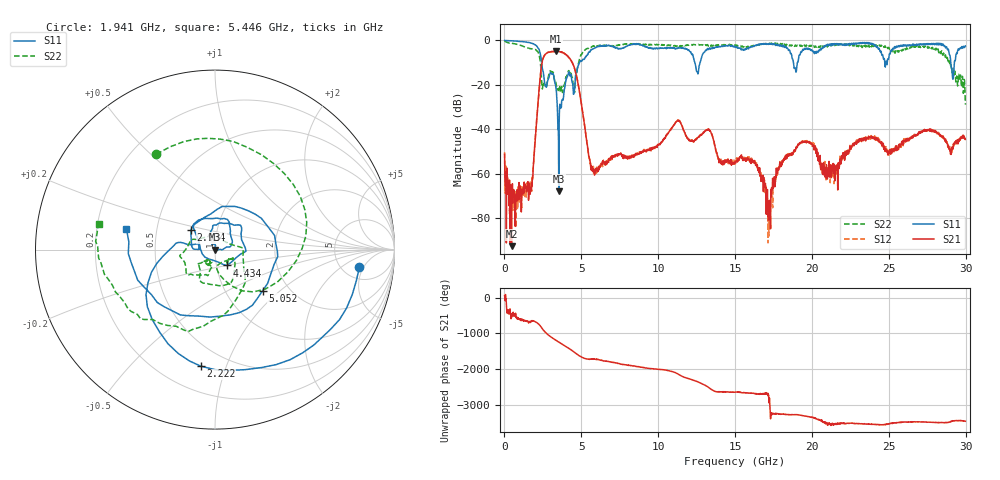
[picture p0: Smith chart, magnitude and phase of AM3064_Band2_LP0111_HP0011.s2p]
# Hz S DB R 50.0
!freq dBS11 angS11 dBS21 angS21 dBS12 angS12 dBS22 angS22
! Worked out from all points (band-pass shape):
!   1600 points, 10 MHz to 29.98 GHz, reference 50 ohm
!   highest |S21| = -4.79 dB at 3.328 GHz (marker M1); lowest = -92.8 dB at 459.8 MHz (marker M2)
!   |S21| within 3 dB of the highest: 2.53 GHz to 4.202 GHz (1.671 GHz wide, 49.6 % of centre)
!   lowest |S11| = -68.0 dB at 3.534 GHz (marker M3), VSWR 1.00, Z = 50 + j0.0316 ohm
!   |S11| at or under -10 dB: 2.416 GHz to 4.88 GHz (2.464 GHz wide, 67.5 % of centre); 12.38 GHz to 12.72 GHz (343.5 MHz wide, 2.74 % of centre); 18.8 GHz to 19.05 GHz (252.6 MHz wide, 1.33 % of centre)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
!   |S22| runs from -28.9 to -0.2 dB; largest |S21 - S12| = 0.023
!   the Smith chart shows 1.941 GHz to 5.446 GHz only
!   S11 on the Smith chart (normalised r, x): 1.941 GHz: 7.17, -4.08; 2.222 GHz: 0.36, -0.82; 2.934 GHz: 0.75, +0.17; 4.434 GHz: 1.12, -0.20; 5.052 GHz: 1.48, -0.78; 5.446 GHz: 0.33, +0.10
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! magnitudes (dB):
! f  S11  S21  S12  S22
! 10 MHz  0.0  -51.3  -50.5  -0.2
! 459.8 MHz  -0.2  -92.8  -71.3  -1.2
! 1.697 GHz  -1.1  -66.1  -66.4  -3.7
! 1.941 GHz  -1.8  -50.4  -50.9  -4.1
! 2.222 GHz  -3.7  -24.9  -24.8  -5.8
! 2.934 GHz  -15.3  -5.3  -5.2  -14.1
! 3.328 GHz  -20.4  -4.8  -4.9  -18.4
! 3.534 GHz  -68.0  -5.0  -5.0  -21.7
! 4.434 GHz  -19.2  -10.3  -10.4  -17.4
! 5.015 GHz  -9.4  -29.1  -28.9  -6.4
! 5.052 GHz  -9.1  -30.7  -30.8  -5.8
! 5.446 GHz  -5.9  -50.0  -50.5  -3.6
! 10 GHz  -3.6  -47.0  -47.0  -2.0
! 11.31 GHz  -3.2  -36.3  -36.2  -2.7
! 15 GHz  -2.7  -54.5  -54.8  -2.0
! 17.2 GHz  -1.6  -76.2  -88.2  -1.6
! 18.06 GHz  -2.1  -55.2  -56.0  -1.9
! 19.99 GHz  -4.4  -46.7  -46.6  -2.2
! 21.04 GHz  -1.8  -61.0  -59.4  -2.1
! 25 GHz  -8.0  -50.1  -49.6  -3.1
! 28.31 GHz  -1.7  -42.9  -43.0  -4.6
! 29.98 GHz  -2.5  -44.6  -43.6  -28.9
